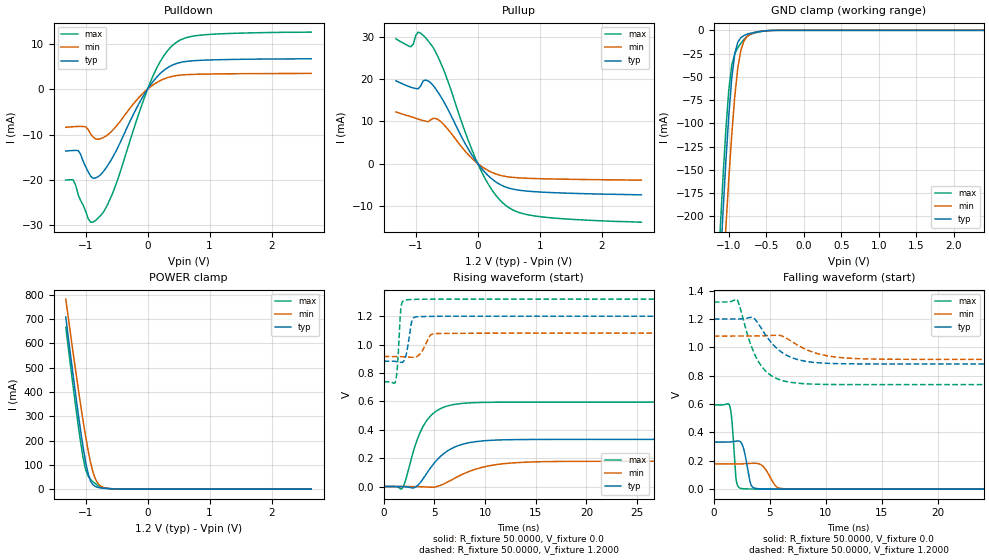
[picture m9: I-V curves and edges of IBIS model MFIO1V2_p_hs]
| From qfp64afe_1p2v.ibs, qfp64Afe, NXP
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[Model] MFIO1V2_p_hs
|   Model MFIO1V2_p_hs
| This model was characterised for following simulation conditions:
| External (pad) voltage:
|   - Typ: 1.2V,   - Min: 1.08V,   - Max: 1.32V
| Library cells for typ/min/max conditions are connected as defined below:
|  IO - External Pad
|  A - Core Input
|  EN - Output Buffer Enable
|  BOOST - vdde
|  EHS - vdd
|  ENZI - vdd
|  EPD - gnd
|  EPUN - vdd
|  ZI - NC
|  ZIF - NC
|  gnd - gnd
|  gnde - gnde
|  vdd - vdd
|  vdde - vdde
| All other pins connected to ground
Model_type I/O
Polarity   Non-Inverting
Enable   Active-Low
Vinl =   0.3600V
Vinh =   0.8400V
Vmeas =  0.6000V
Cref =   20.0000F
Rref =   1.0000M
Vref =   0.0V
C_comp   1.6652pF   1.5787pF   1.7428pF
|C_comp_pullup   0.8462pF   0.8814pF   0.7990pF
|C_comp_pulldown   0.6044pF   0.6428pF   0.5687pF
[Model Spec]
| variable   typ   min   max
Vinh   0.3600V   0.3240V   0.3960V
Vinl   0.8400V   0.7560V   0.9240V
Vmeas   0.6000V   0.5400V   0.6600V
[Temperature Range]   25.0000   0.1250k   -40.0000
[Voltage Range]   1.2000V   1.0800V   1.3200V
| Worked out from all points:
|   slope of the pulldown table from 0 to 0.18 V, typ, clamps not added: 58.2 ohm
|   slope of the pullup table from 0 to 0.18 V, typ, clamps not added: 59.4 ohm
|   GND clamp passes 1 mA (typ) near -0.57 V on its own axis
|   POWER clamp passes 1 mA (typ) near -0.54 V on its own axis
|   rising waveform, R_fixture 50.0000, V_fixture 0.0: 20-80 % time 2.65ns typ, 3.74ns min, 1.91ns max; typ from 0 V to 0.332 V
|   rising waveform, R_fixture 50.0000, V_fixture 1.2000: 20-80 % time 420ps typ, 689ps min, 271ps max; typ from 0.883 V to 1.2 V
|   falling waveform, R_fixture 50.0000, V_fixture 0.0: 20-80 % time 470ps typ, 798ps min, 303ps max; typ from 0.332 V to 0 V
|   falling waveform, R_fixture 50.0000, V_fixture 1.2000: 20-80 % time 2.23ns typ, 2.82ns min, 1.78ns max; typ from 1.2 V to 0.883 V
[Pulldown]
|Voltage   I(typ)   I(min)   I(max)
-1.32V    -13.65mA   -8.413mA   -20.02mA
-1.2V     -13.51mA   -8.286mA   -20.01mA
-1.12V    -13.55mA   -8.228mA   -23.23mA
-920mV    -19.16mA   -9.85mA    -29.29mA
-720mV    -18.27mA   -10.7mA    -27.21mA
-520mV    -13.92mA   -8.406mA   -21.33mA
-160mV    -3.727mA   -2.148mA   -6.154mA
80mV      1.535mA    840.4uA    2.681mA
280mV     4.299mA    2.312mA    7.674mA
480mV     5.684mA    2.989mA    10.42mA
960mV     6.383mA    3.3mA      11.99mA
2.64V     6.671mA    3.446mA    12.53mA
[Pullup]
|Voltage   I(typ)   I(min)   I(max)
-1.32V    19.64mA    12.26mA    29.61mA
-1.08V    18.12mA    11.13mA    27.73mA
-960mV    17.74mA    10.54mA    31.21mA
-840mV    19.83mA    10.07mA    29.84mA
-720mV    18.57mA    10.71mA    27.56mA
-520mV    13.94mA    8.794mA    21.09mA
-200mV    4.663mA    2.883mA    7.362mA
40mV      -771.3uA   -452.7uA   -1.28mA
240mV     -3.804mA   -2.171mA   -6.507mA
480mV     -5.732mA   -3.143mA   -10.26mA
1.04V     -6.794mA   -3.614mA   -12.68mA
2.64V     -7.439mA   -3.951mA   -13.93mA
[GND_clamp]
|Voltage   I(typ)   I(min)   I(max)
-1.32V    -596.2mA   -647.7mA   -564.2mA
-1.12V    -261.7mA   -329.6mA   -222.8mA
-1.08V    -200.1mA   -270.2mA   -162.2mA
-1.04V    -142.4mA   -213.4mA   -108mA
-1V       -91.65mA   -160.1mA   -64.39mA
-960mV    -51.25mA   -111.8mA   -37.35mA
-920mV    -25.17mA   -71.04mA   -25.18mA
-880mV    -12.88mA   -40.68mA   -18.84mA
-800mV    -5.691mA   -11.78mA   -10.04mA
-680mV    -2.577mA   -2.919mA   -3.527mA
-440mV    -153.3uA   -179.9uA   -188.4uA
2.64V     0A         0A         0A
[POWER_clamp]
|Voltage   I(typ)   I(min)   I(max)
-1.32V    708.1mA    782.2mA    666.5mA
-1.2V     465.4mA    558mA      418.6mA
-1.12V    311.6mA    414.7mA    262.8mA
-1.04V    171.5mA    279.6mA    128mA
-1V       111.6mA    216.9mA    80.26mA
-960mV    64.04mA    159.3mA    53.83mA
-920mV    32.99mA    108.8mA    40.2mA
-880mV    17.4mA     68.42mA    30.38mA
-840mV    10.74mA    40.16mA    22.02mA
-760mV    5.263mA    13.19mA    9.321mA
-440mV    204.8uA    279.1uA    238.1uA
2.64V     0A         0A         0A
[Ramp]
| variable   typ   min   max
dV/dt_r  0.1990/2.6510n   0.1067/3.7402n   0.3565/1.9134n
dV/dt_f  0.1903/2.2318n   98.6896m/2.8167n   0.3495/1.7771n
R_load = 50.0000
[Rising Waveform]
R_fixture= 50.0000
V_fixture= 0.0
V_fixture_min= 0.0
V_fixture_max= 0.0
|time   V(typ)   V(min)   V(max)
0s        1.255nV    120.3nV    51.27pV
1.855ns   -190.2uV   79.91uV    -9.107mV
2.173ns   -1.996mV   82uV       46.62mV
3.369ns   8.594mV    -694.9uV   341.8mV
4.618ns   130.9mV    -5.217mV   497mV
5.982ns   234.9mV    19.74mV    559.8mV
7.943ns   300.6mV    91.62mV    586.5mV
11.2ns    327.3mV    155.2mV    593.6mV
16.07ns   331.6mV    175.4mV    594.1mV
100ns     331.7mV    177.8mV    594.1mV
[Rising Waveform]
R_fixture= 50.0000
V_fixture= 1.2000
V_fixture_min= 1.0800
V_fixture_max= 1.3200
|time   V(typ)   V(min)   V(max)
0s        882.9mV    915.5mV    737.5mV
1.17ns    880.9mV    915.8mV    740.6mV
1.354ns   878.5mV    915.9mV    841.3mV
1.729ns   873.6mV    914.7mV    1.27V
2.146ns   909.6mV    912.7mV    1.313V
2.549ns   1.068V     910.7mV    1.316V
2.985ns   1.19V      909.8mV    1.318V
4.59ns    1.198V     1.064V     1.319V
5.393ns   1.199V     1.078V     1.32V
100ns     1.2V       1.08V      1.32V
[Falling Waveform]
R_fixture= 50.0000
V_fixture= 0.0
V_fixture_min= 0.0
V_fixture_max= 0.0
|time   V(typ)   V(min)   V(max)
0s        331.7mV    177.8mV    594.1mV
1.417ns   332.1mV    177.8mV    589.3mV
1.617ns   334mV      177.7mV    484.9mV
2.013ns   339.1mV    177.6mV    59.11mV
2.599ns   302.2mV    178.9mV    3.084mV
3.31ns    34.2mV     182.1mV    1.137mV
4.18ns    2.166mV    173.7mV    484.6uV
5.59ns    632uV      17.07mV    143.3uV
6.699ns   290.5uV    1.725mV    58.66uV
100ns     2.852nV    124.9nV    7.782nV
[Falling Waveform]
R_fixture= 50.0000
V_fixture= 1.2000
V_fixture_min= 1.0800
V_fixture_max= 1.3200
|time   V(typ)   V(min)   V(max)
0s        1.2V       1.08V      1.32V
2.05ns    1.2V       1.08V      1.34V
2.27ns    1.2V       1.08V      1.301V
3.488ns   1.211V     1.08V      980.5mV
4.368ns   1.119V     1.081V     855.8mV
5.86ns    977.1mV    1.085V     772.9mV
7.896ns   906.6mV    998mV      744.8mV
10.35ns   887.1mV    937.6mV    738.4mV
15.19ns   883mV      916.7mV    737.4mV
100ns     882.9mV    915.5mV    737.5mV
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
